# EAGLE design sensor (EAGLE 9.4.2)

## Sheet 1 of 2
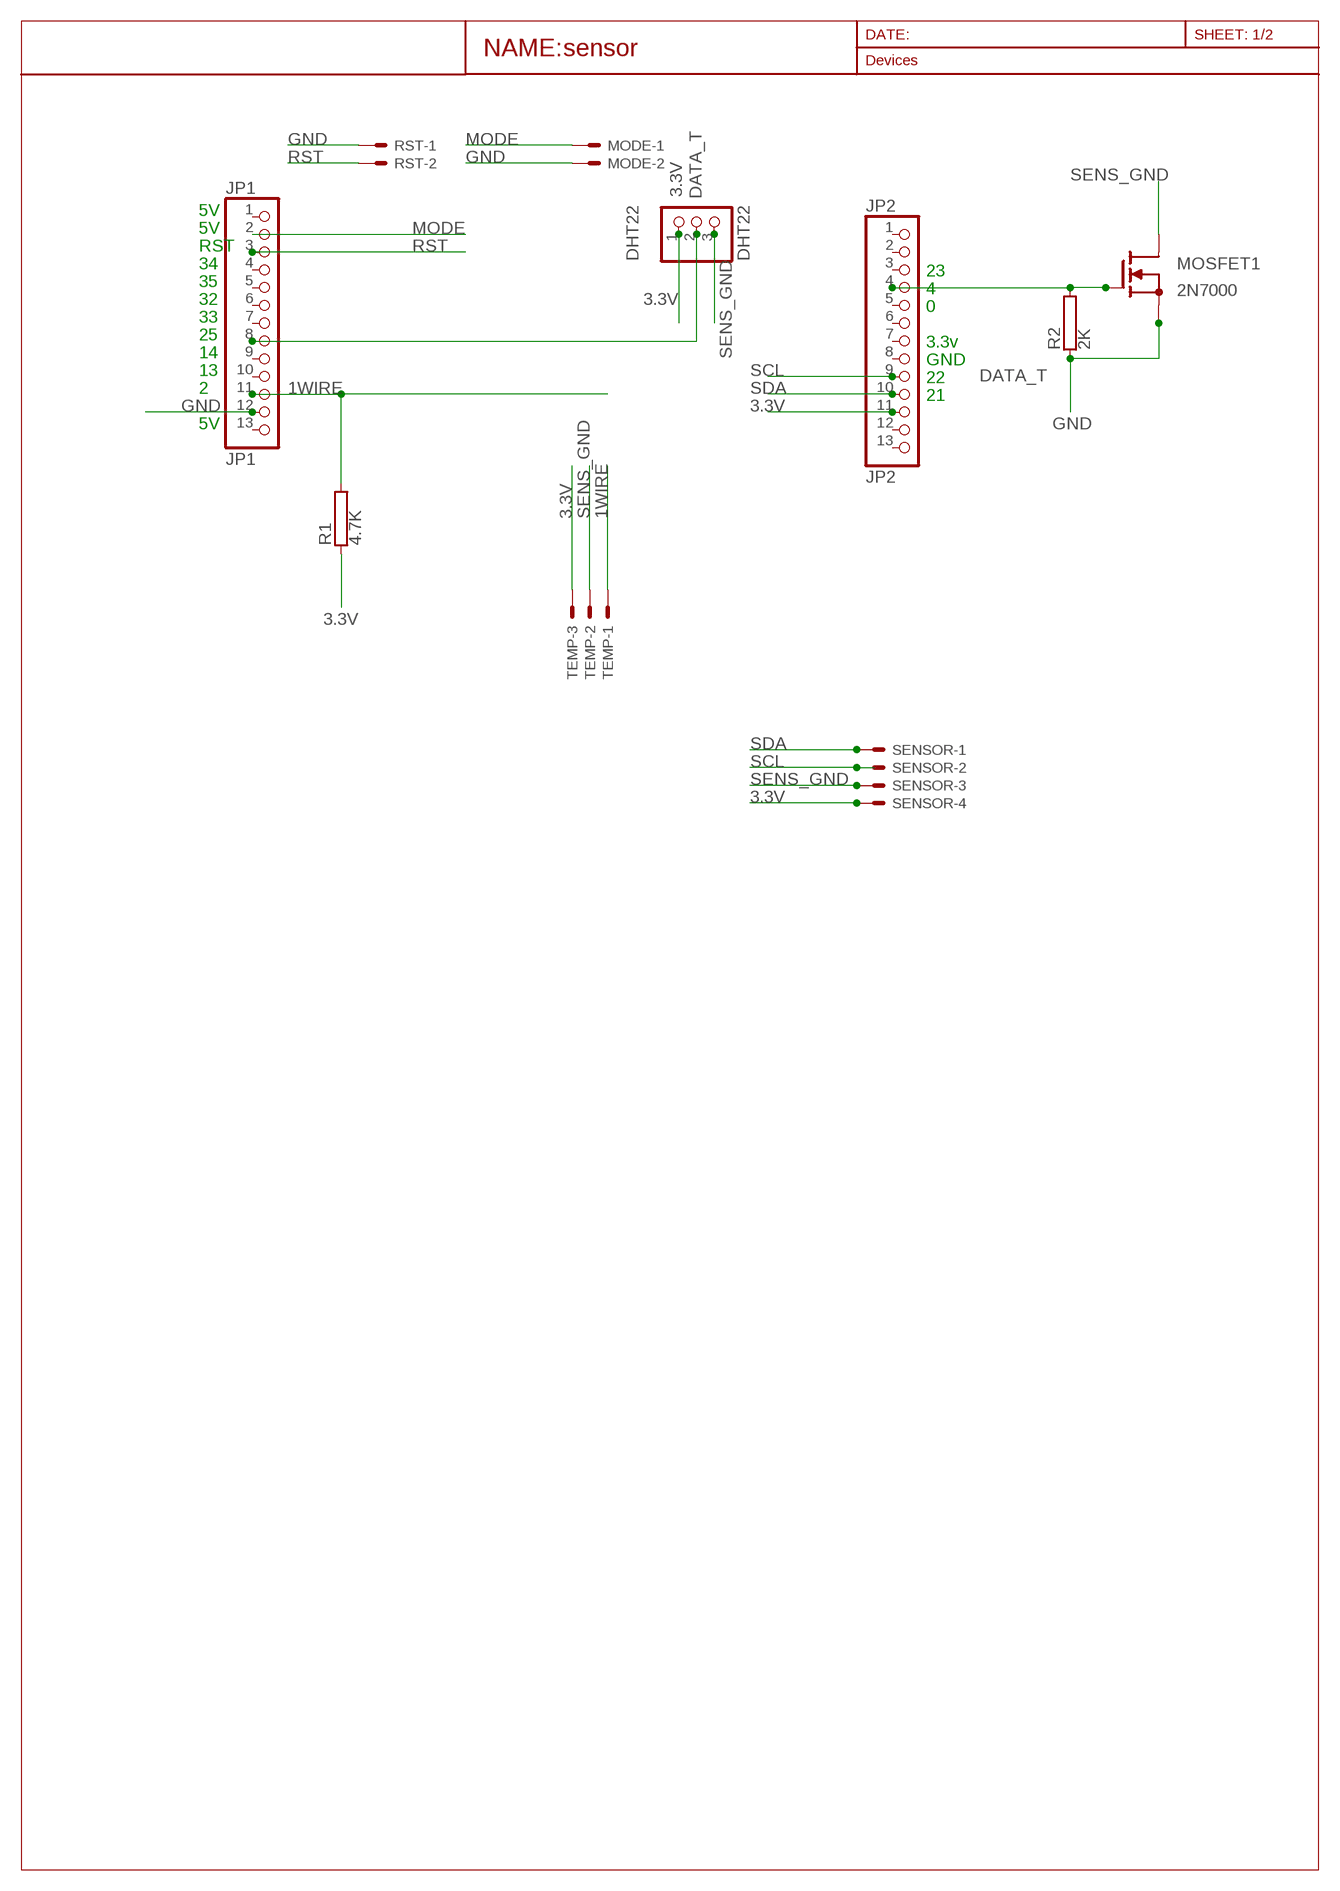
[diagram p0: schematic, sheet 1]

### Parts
DHT22  DHT22  PINHD-1X3  [1X03]
JP1  JP1  PINHD-1X13  [1X13]
JP2  JP2  PINHD-1X13  [1X13]
MODE  JST-XH-02-PIN-LONG-PAD  [JST-XH-02-PACKAGE-LONG-PAD]
MOSFET1  2N7000  [TO92]
R1  4.7K  RHPS58  [HPS58]
R2  2K  RHPS58  [HPS58]
RST  JST-XH-02-PIN-LONG-PAD  [JST-XH-02-PACKAGE-LONG-PAD]
SENSOR  JST-XH-04-PIN-LONG-PAD  [JST-XH-04-PACKAGE-LONG-PAD]
TEMP  JST-XH-03-PIN-LONG-PAD  [JST-XH-03-PACKAGE-LONG-PAD]

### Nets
1WIRE [pwr]: JP1.11 R1.2 TEMP.1
3.3V [pwr]: DHT22.1 JP2.11 R1.1 SENSOR.4 TEMP.3
DATA_T [pwr]: DHT22.2 JP1.8
GND [pwr]: JP1.12 MODE.2 MOSFET1.C(S) R2.1 RST.1
MODE [pwr]: JP1.2 MODE.1
RST [pwr]: JP1.3 RST.2
SCL [pwr]: JP2.9 SENSOR.2
SDA [pwr]: JP2.10 SENSOR.1
SENS_ENABLE [pwr]: JP2.4 MOSFET1.B(G) R2.2
SENS_GND [pwr]: DHT22.3 MOSFET1.E(D) SENSOR.3 TEMP.2
Unconnected: JP1.1 JP1.4 JP1.5 JP1.6 JP1.7 JP1.9 JP1.10 JP1.13 JP2.1 JP2.2 JP2.3 JP2.5 JP2.6 JP2.7 JP2.8 JP2.12 JP2.13

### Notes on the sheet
- 5V
- 5V
- RST
- 34
- 23
- 35
- 4
- 32
- 0
- 33
- 25
- 3.3v
- 14
- GND
- 13
- 22
- 2
- 21
- 5V

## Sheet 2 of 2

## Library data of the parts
DHT22 = adafruit:PINHD-1X3: PIN HEADER
JP1 JP2 = adafruit:PINHD-1X13: PIN HEADER
MODE RST = Rembrandt Electronics - JST XH Connectors v1-0:JST-XH-02-PIN: JST XH Connector 2 Pin
MOSFET1 = 2N7000:2N7000; AVAILABILITY: Unavailable; DESCRIPTION: MOSFETs- Power and Small Signal 60V 200mA N-Channel No-Cancel/No-Return; MF: STMicroelectronics; MP: 2N7000; PACKAGE: TO-92 ON Semiconductor; PRICE: None
R1 R2 = resistor-power:R: Power Resitor; OC_FARNELL: unknown; OC_NEWARK: unknown
SENSOR = Rembrandt Electronics - JST XH Connectors v1-0:JST-XH-04-PIN: JST XH Connector 2 Pin Wire to board connector. Pitch: 2,54 mm, (0.100") Number of pins: 4 Created by Rembrandt Electronics www.rembrandtelectronics.com
TEMP = Rembrandt Electronics - JST XH Connectors v1-0:JST-XH-03-PIN: JST XH Connector 2 Pin Wire to board connector. Pitch: 2,54 mm, (0.100") Number of pins: 3 Created by Rembrandt Electronics www.rembrandtelectronics.com

## Module SWITCHES
Ports: 

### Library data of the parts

## Module POWER
Ports: VCC(io) 3.3V(io) GND(io) ENABLE(io)

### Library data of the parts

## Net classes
1 pwr: width 0.6 mm

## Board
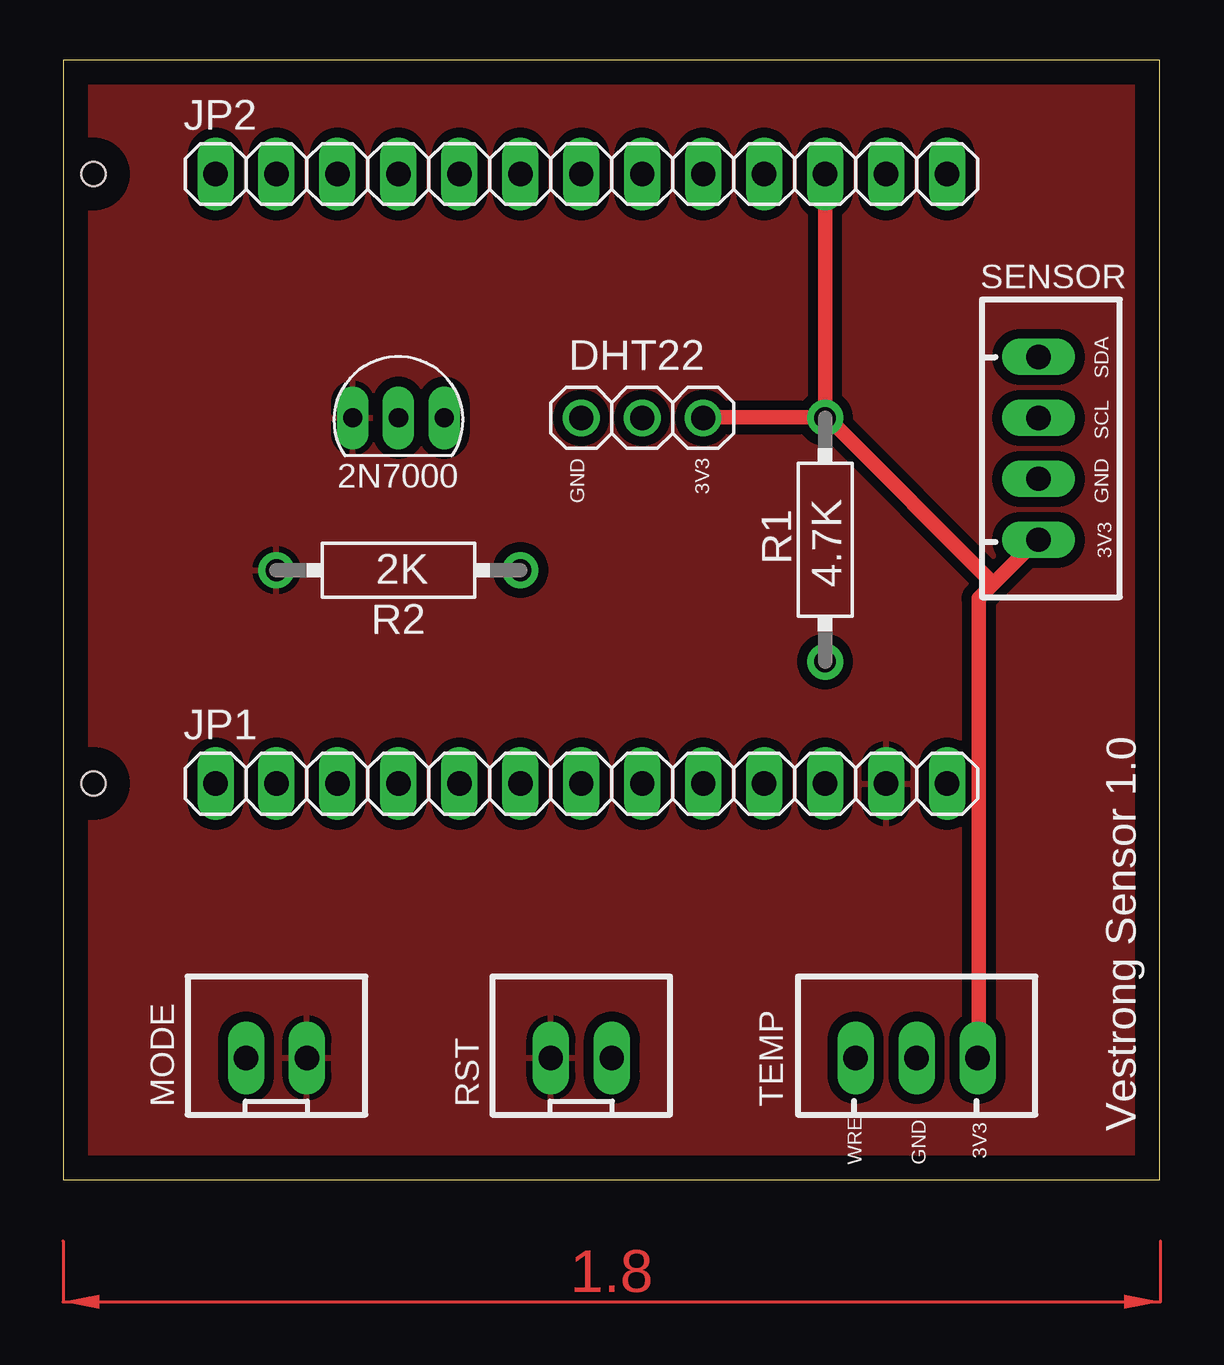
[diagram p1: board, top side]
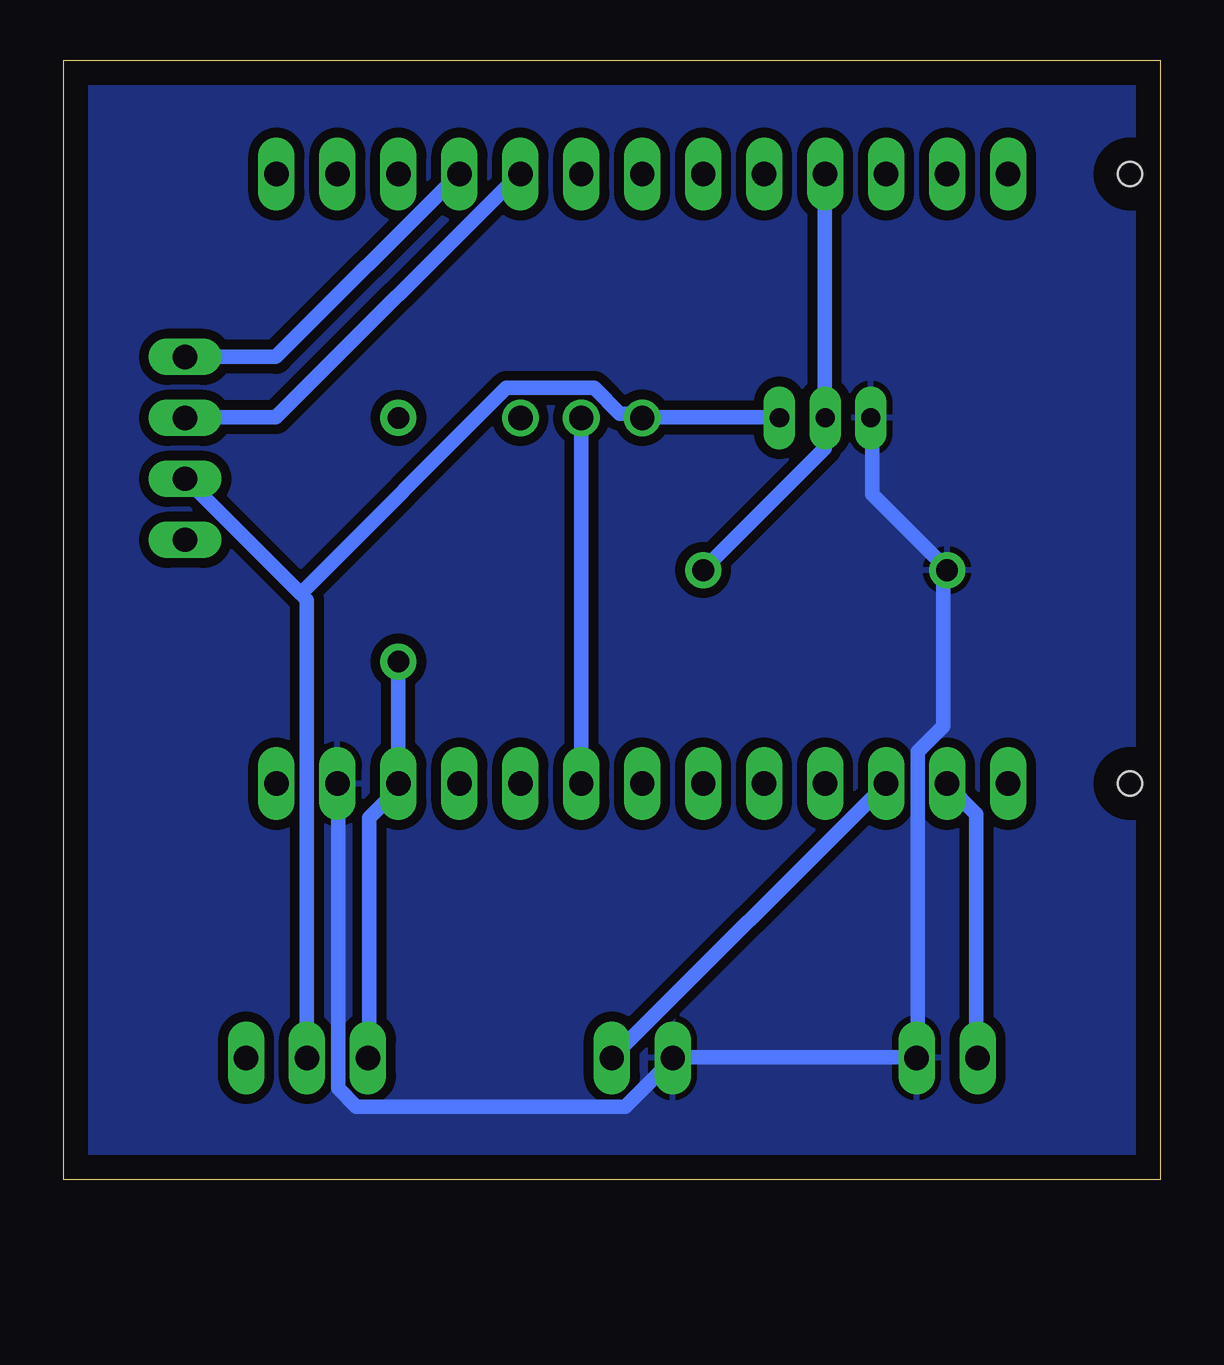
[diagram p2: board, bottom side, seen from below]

Size 45.7 x 46.66 mm. Coordinates in mm from the lower left corner, seen from the top.
Outline: 0,0 45.7,0 45.7,46.66 0,46.66 0,0
Copper layers (1*16): Top 0.035mm / dielectric 1.5mm / Bottom 0.035mm
Design rules "default": minimum track width 6mil, minimum drill 0.35mm, track to track 6mil, track to pad 6mil, pad to pad 6mil, via to via 6mil, smd to smd 6mil, copper to edge 40mil, drill to drill 6mil, minimum pad ring 10mil, minimum via ring 8mil, stop-mask expansion 4mil, vias tented up to drill 0mil, thermal gap 10mil
Holes 1 mm at 1.27,16.51 1.27,41.91

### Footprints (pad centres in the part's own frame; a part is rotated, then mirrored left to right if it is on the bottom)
1X03 = drill 1.016: 1 -2.54,0; 2 0,0; 3 2.54,0
1X13 = drill 1.016 long: 1 -15.24,0; 2 -12.7,0; 3 -10.16,0; 4 -7.62,0; 5 -5.08,0; 6 -2.54,0; 7 0,0; 8 2.54,0; 9 5.08,0; 10 7.62,0; 11 10.16,0; 12 12.7,0; 13 15.24,0
JST-XH-02-PACKAGE-LONG-PAD = drill 1.016 long: 1 -1.27,0; 2 1.27,0
TO92 = drill 0.8 pad 1.27 long: B 0,0; C 0,-1.905; E 0,1.905
HPS58 = drill 0.9 pad 1.5: 1 -5.08,0; 2 5.08,0
JST-XH-04-PACKAGE-LONG-PAD = drill 1.016 long: 1 -3.81,0; 2 -1.27,0; 3 1.27,0; 4 3.81,0
JST-XH-03-PACKAGE-LONG-PAD = drill 1.016 long: 1 -2.54,0; 2 0,0; 3 2.54,0

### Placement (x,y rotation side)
DHT22  24.13,31.75 180 top
JP1  21.59,16.51 0 top
JP2  21.59,41.91 0 top
MODE  8.89,5.08 0 top
MOSFET1  13.97,31.75 270 top
R1  31.75,26.67 270 top
R2  13.97,25.4 0 top
RST  21.59,5.08 0 top
SENSOR  40.64,30.48 270 top
TEMP  35.56,5.08 0 top

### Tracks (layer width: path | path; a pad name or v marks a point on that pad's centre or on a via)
1WIRE
  Bottom 0.6: R1.2 JP1.11 31.83,16.23 32.97,15.09 32.97,5.11 TEMP.1
3.3V
  Top 0.6: R1.1 31.75,31.77 26.72,31.77 DHT22.1 | R1.1 JP2.11 | 38.76,24.84 40.59,26.67 SENSOR.4 | 38.76,24.84 38.15,24.23 38.15,5.11 TEMP.3 | 38.76,24.84 31.98,31.62 R1.1
DATA_T
  Bottom 0.6: DHT22.2 JP1.8
GND
  Bottom 0.6: MOSFET1.C 12.01,31.7 12.01,28.57 8.89,25.45 R2.1 9.04,25.15 9.04,18.9 10.11,17.83 10.11,5.33 MODE.2 10.19,5.11 20.32,5.11 RST.1 20.47,4.88 22.3,3.05 33.5,3.05 34.27,3.81 34.27,16.46 JP1.12
  pour Bottom (isolate 0.406): 0,0 0,46.99 45.72,46.99 45.72,0
  pour Top (isolate 0.406): 0,46.99 45.72,46.99 45.72,0 0,0
MODE
  Bottom 0.6: MODE.1 7.67,5.11 7.67,15.24 8.89,16.46 JP1.2
RST
  Bottom 0.6: JP1.3 RST.2
SCL
  Bottom 0.6: SENSOR.2 40.59,31.77 36.85,31.77 26.72,41.91 JP2.9
SDA
  Bottom 0.6: SENSOR.1 36.85,34.29 29.23,41.91 JP2.10
SENS_ENABLE
  Bottom 0.6: R2.2 19.02,25.45 13.99,30.48 13.99,31.7 MOSFET1.B 13.99,32 13.99,41.91 JP2.4
SENS_GND
  Bottom 0.6: MOSFET1.E 15.9,31.77 21.54,31.77 DHT22.3 21.84,31.93 22.53,31.93 23.6,32.99 27.25,32.99 35.83,24.42 | TEMP.2 35.56,24.16 35.83,24.42 | 35.83,24.42 40.59,29.18 SENSOR.3
(copper drawn outside any net)
  shapes: Top area x2

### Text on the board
tPlace: SDA | SCL | 3V3 | GND | GND | 3V3 | Vestrong Sensor 1.0 | WRE | GND | 3V3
